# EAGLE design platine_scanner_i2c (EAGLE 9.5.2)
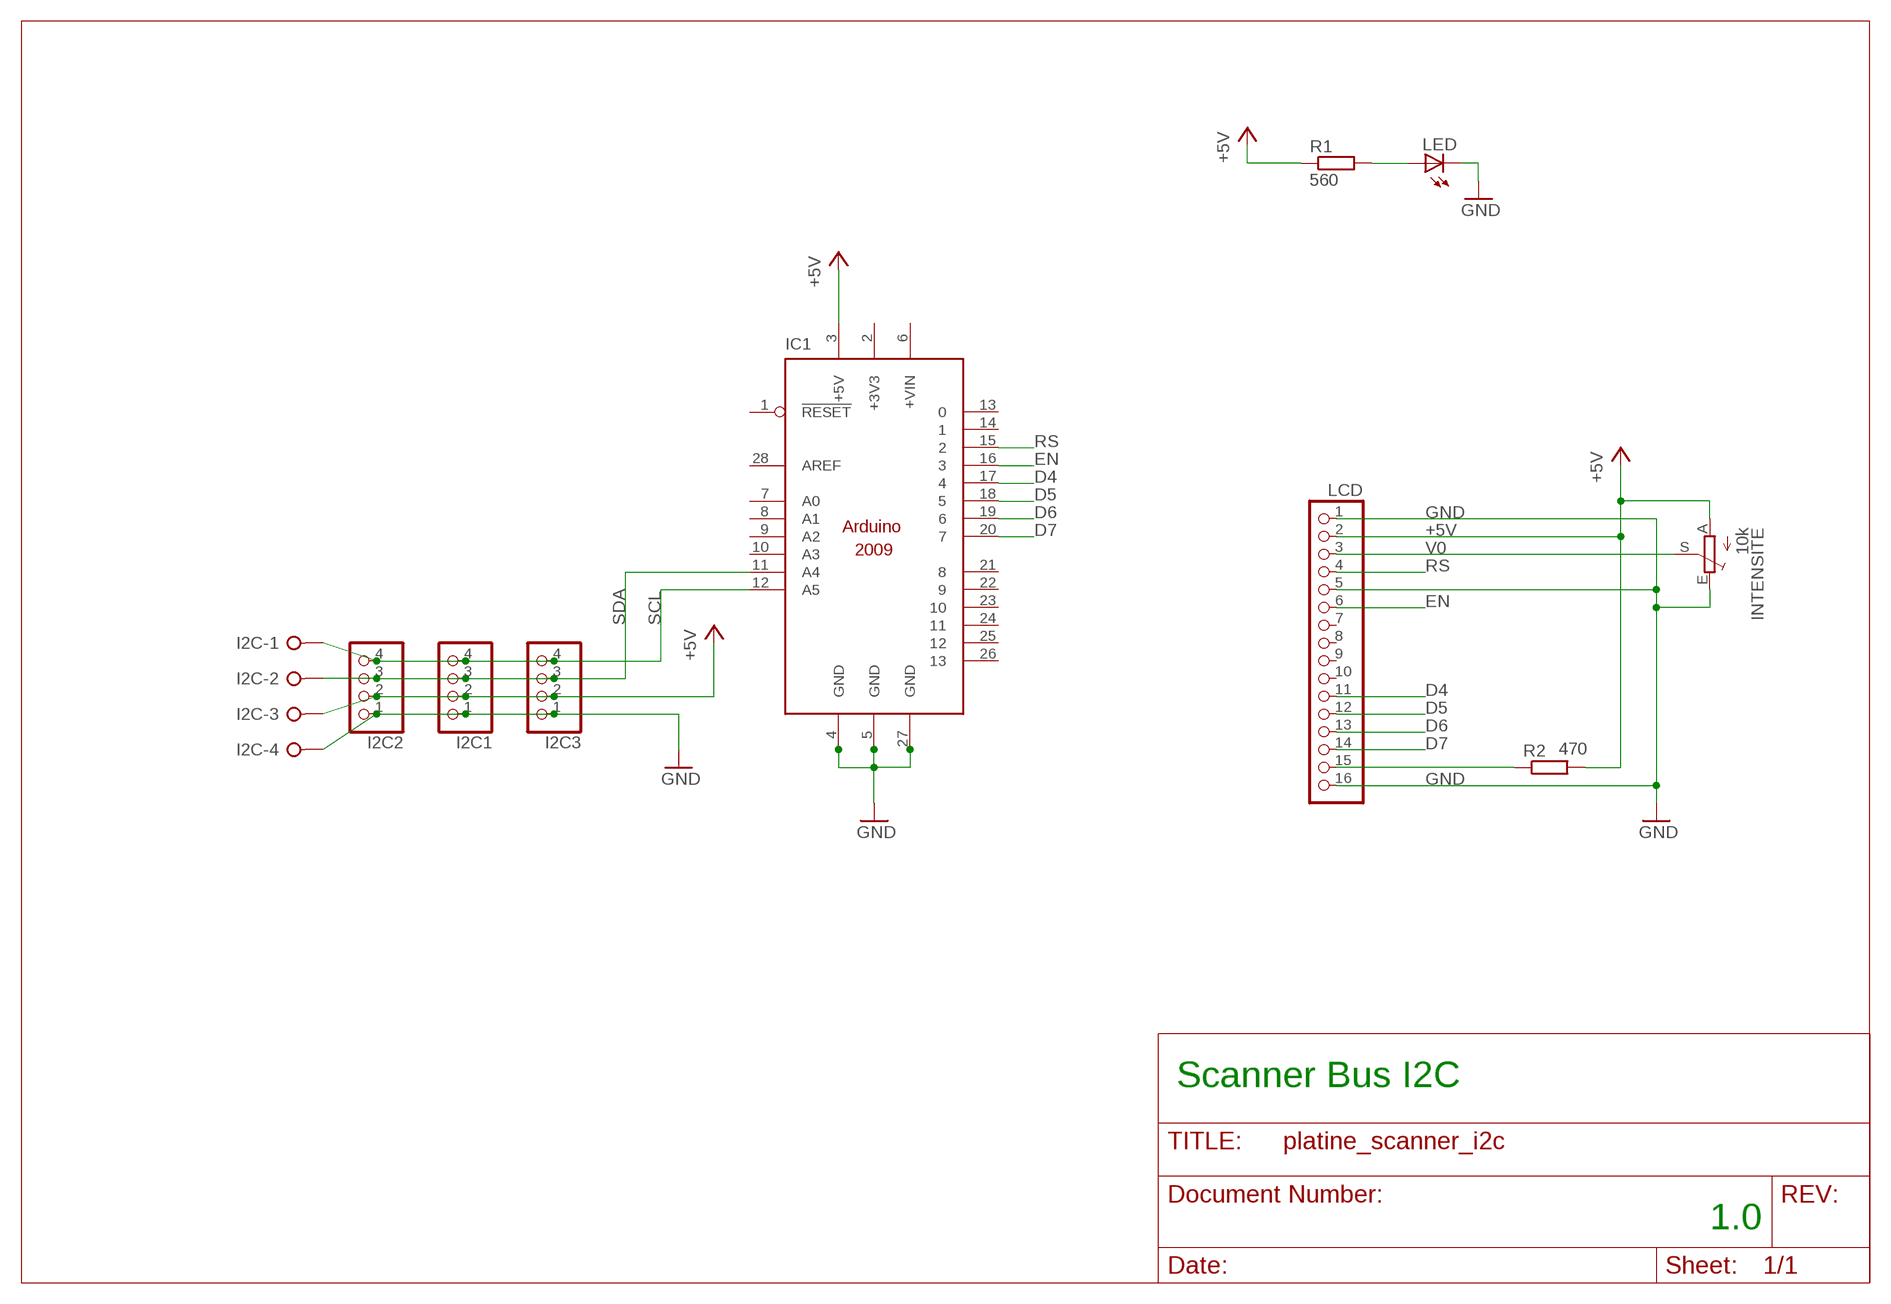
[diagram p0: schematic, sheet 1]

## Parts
I2C  W237-04P  [W237-4P]
I2C1  PINHD-1X4  [1X04]
I2C2  PINHD-1X4  [1X04]
I2C3  PINHD-1X4  [1X04]
IC1  ARDUINO2009_11  [ARDUINO2009_1]
INTENSITE  10k  TRIM_EU-LI10  [LI10]
LCD  PINHD-1X16  [1X16]
LED  LED3MM  [LED3MM]
R1  560  R-EU_0204/7  [0204/7]
R2  470  R-EU_0204/7  [0204/7]

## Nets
+5V: I2C1.2 I2C2.2 I2C3.2 I2C.3 IC1.3(+5V) INTENSITE.A LCD.2 R1.1 R2.2
D4: IC1.17 LCD.11
D5: IC1.18 LCD.12
D6: IC1.19 LCD.13
D7: IC1.20 LCD.14
EN: IC1.16 LCD.6
GND: I2C1.1 I2C2.1 I2C3.1 I2C.4 IC1.4(GND) IC1.5(GND) IC1.27(GND) INTENSITE.E LCD.1 LCD.5 LCD.16 LED.K(C)
N$1: LED.A R1.2
N$15: LCD.15 R2.1
RS: IC1.15 LCD.4
SCL: I2C1.4 I2C2.4 I2C3.4 I2C.1 IC1.12(A5)
SDA: I2C1.3 I2C2.3 I2C3.3 I2C.2 IC1.11(A4)
V0: INTENSITE.S LCD.3
Unconnected: IC1.1(!RESET) IC1.6(+VIN) IC1.7(A0) IC1.8(A1) IC1.9(A2) IC1.10(A3) IC1.13 IC1.14 IC1.21 IC1.22 IC1.23 IC1.24 IC1.25 IC1.26 IC1.28(AREF) LCD.7 LCD.8 LCD.9 LCD.10

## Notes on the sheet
- Scanner Bus I2C
- 1.0

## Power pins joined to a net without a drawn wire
+3V3: IC1.2(+3V3)

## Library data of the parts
I2C = con-wago-508:W237-04P: WAGO SREW CLAMP; OC_FARNELL: unknown; OC_NEWARK: unknown
I2C1-I2C3 = pinhead:PINHD-1X4: PIN HEADER
IC1 = arduino_uno:ARDUINO2009_1: The Arduino Duemilanove ("2009") is a microcontroller board based on the ATmega168 or ATmega328. - 14 digital input/output pins (of which 6 can be used as PWM outputs) - 6 analog inputs, a 16 MHz crystal oscillator - USB connection - power jack - ISP header - reset button It contains everything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
INTENSITE = pot:TRIM_EU-: POTENTIOMETER
LCD = pinhead:PINHD-1X16: PIN HEADER
LED = led:LED: LED
R1 R2 = rcl:R-EU_: RESISTOR, European symbol

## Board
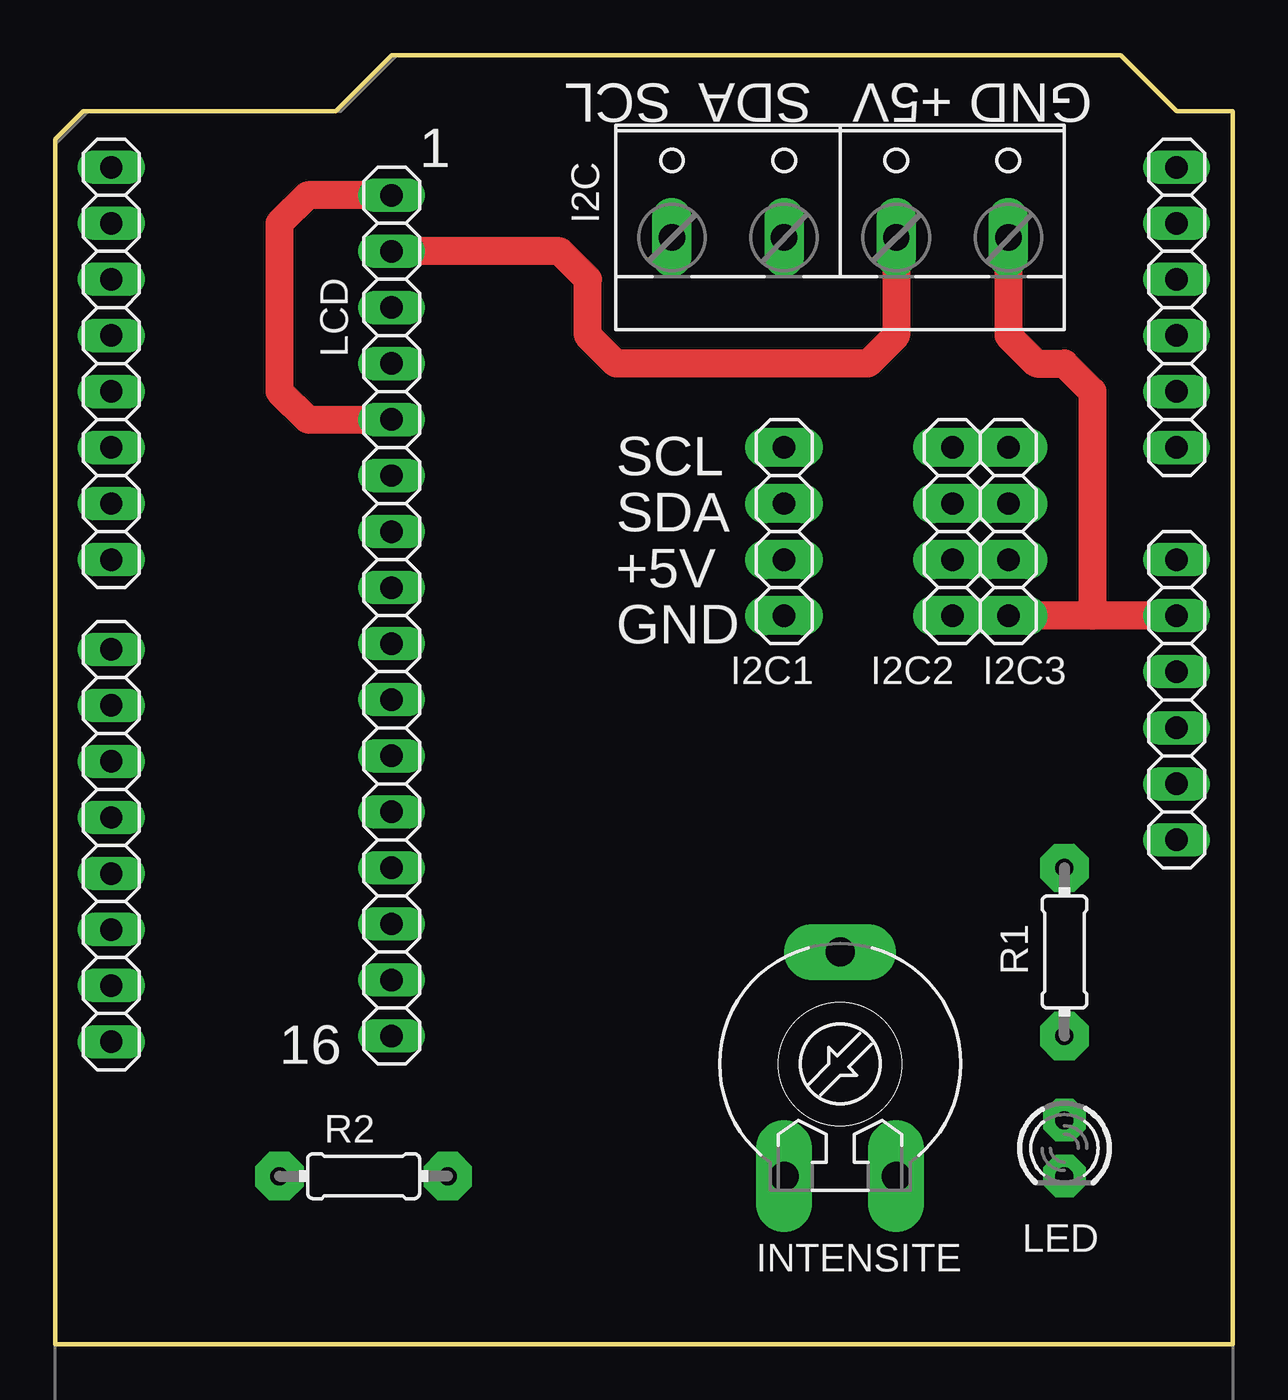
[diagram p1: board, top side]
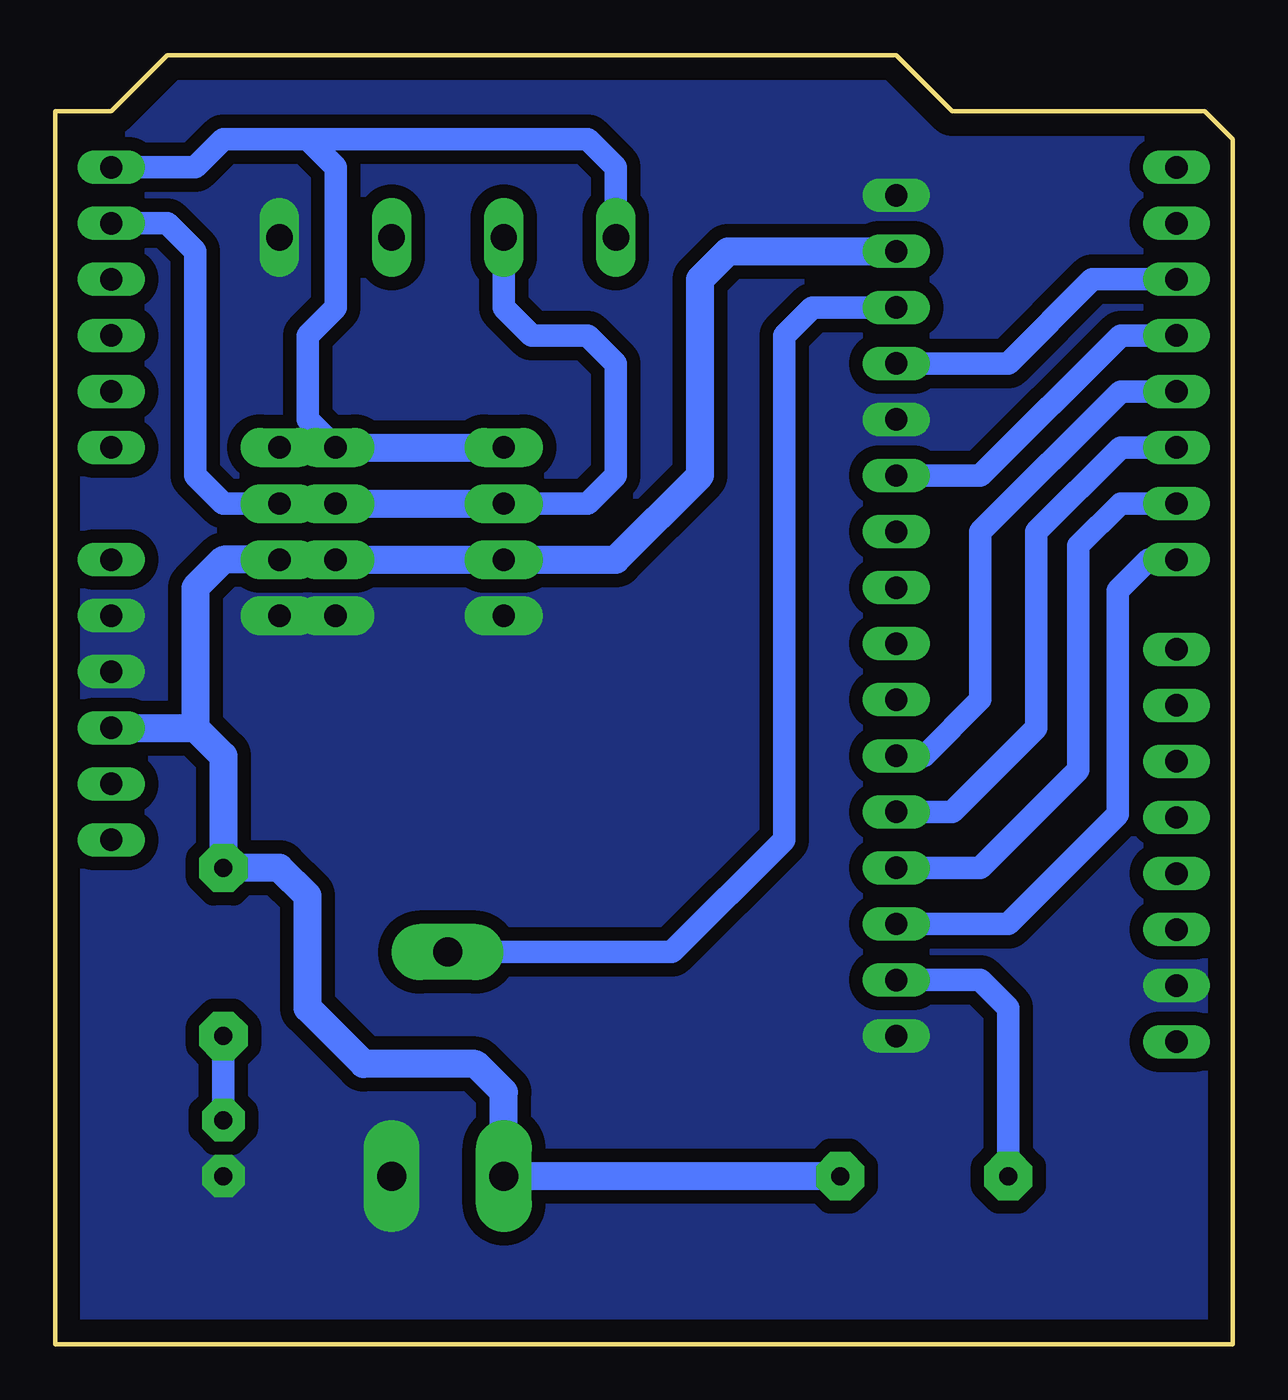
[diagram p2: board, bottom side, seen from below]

Size 53.34 x 58.42 mm. Coordinates in mm from the lower left corner, seen from the top.
Outline: 0,0 0,54.61 1.27,55.88 12.7,55.88 15.24,58.42 48.26,58.42 50.8,55.88 53.34,55.88 53.34,0 0,0
Copper layers (1*16): Top 0.035mm / dielectric 1.5mm / Bottom 0.035mm
Design rules "default": minimum track width 6mil, minimum drill 0.35mm, track to track 6mil, track to pad 6mil, pad to pad 6mil, via to via 6mil, smd to smd 6mil, copper to edge 40mil, drill to drill 6mil, minimum pad ring 10mil, minimum via ring 8mil, stop-mask expansion 4mil, vias tented up to drill 0mil, thermal gap 10mil

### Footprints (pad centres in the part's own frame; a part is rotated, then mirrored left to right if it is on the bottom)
W237-4P = drill 1.194 long: 1 -7.62,-0.635; 2 -2.54,-0.635; 3 2.54,-0.635; 4 7.62,-0.635
1X04 = drill 1.016 pad 1.778 long: 1 -3.81,0; 2 -1.27,0; 3 1.27,0; 4 3.81,0
ARDUINO2009_1 = drill 1.016 long: 1 33.02,2.54; 2 35.56,2.54; 3 38.1,2.54; 4 40.64,2.54; 5 43.18,2.54; 6 45.72,2.54; 7 50.8,2.54; 8 53.34,2.54; 9 55.88,2.54; 10 58.42,2.54; 11 60.96,2.54; 12 63.5,2.54; 13 63.5,50.8; 14 60.96,50.8; 15 58.42,50.8; 16 55.88,50.8; 17 53.34,50.8; 18 50.8,50.8; 19 48.26,50.8; 20 45.72,50.8; 21 41.656,50.8; 22 39.116,50.8; 23 36.576,50.8; 24 34.036,50.8; 25 31.496,50.8; 26 28.956,50.8; 27 26.416,50.8; 28 23.876,50.8
LI10 = drill 1.321 pad 2.54 long: A -2.54,-5.08; E 2.54,-5.08; S 0,5.08
1X16 = drill 1.016 long: 1 -19.05,0; 2 -16.51,0; 3 -13.97,0; 4 -11.43,0; 5 -8.89,0; 6 -6.35,0; 7 -3.81,0; 8 -1.27,0; 9 1.27,0; 10 3.81,0; 11 6.35,0; 12 8.89,0; 13 11.43,0; 14 13.97,0; 15 16.51,0; 16 19.05,0
LED3MM = drill 0.813 pad 1.93 octagon: A -1.27,0; K 1.27,0
0204/7 = drill 0.813 pad 2.184 octagon: 1 -3.81,0; 2 3.81,0

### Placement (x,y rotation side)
I2C  35.56,50.8 0 top
I2C1  33.02,36.83 90 top
I2C2  43.18,36.83 90 top
I2C3  40.64,36.83 90 top
IC1  53.34,-10.16 90 top
INTENSITE  35.56,12.7 0 top
LCD  15.24,33.02 270 top
LED  45.72,8.89 270 top
R1  45.72,17.78 270 top
R2  13.97,7.62 0 top

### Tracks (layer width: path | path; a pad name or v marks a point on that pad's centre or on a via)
+5V
  Top 1.27: I2C.3 38.1,45.72 36.83,44.45 25.4,44.45 24.13,45.72 24.13,48.26 22.86,49.53 LCD.2
  Bottom 1.27: 46.99,27.94 45.72,26.67 R1.1 43.18,21.59 41.91,20.32 41.91,15.24 39.37,12.7 34.29,12.7 33.02,11.43 INTENSITE.A R2.2 | LCD.2 22.86,49.53 24.13,48.26 24.13,39.37 27.94,35.56 I2C1.2 I2C3.2 I2C2.2 45.72,35.56 46.99,34.29 46.99,27.94 | IC1.3 46.99,27.94
D4
  Bottom 1.016: LCD.11 13.97,26.67 11.43,29.21 11.43,36.83 5.08,43.18 IC1.17
D5
  Bottom 1.016: LCD.12 12.7,24.13 8.89,27.94 8.89,36.83 5.08,40.64 IC1.18
D6
  Bottom 1.016: IC1.19 5.08,38.1 6.98,36.2 6.98,26.04 11.43,21.59 LCD.13
D7
  Bottom 1.016: LCD.14 10.16,19.05 5.21,24 5.21,34.16 3.81,35.56 IC1.20
EN
  Bottom 1.016: IC1.16 5.08,45.72 11.43,39.37 LCD.6
GND
  Top 1.27: I2C.4 43.18,45.72 44.45,44.45 45.72,44.45 46.99,43.18 46.99,33.02 I2C2.1 IC1.5 | LCD.5 11.43,41.91 10.16,43.18 10.16,50.8 11.43,52.07 LCD.1
  pour Bottom (isolate 0.61, no thermals): -1.27,58.42 -1.27,-1.27 54.61,-1.27 54.61,58.42
N$1
  Bottom 1.016: R1.2 LED.A
N$15
  Bottom 1.016: LCD.15 11.43,16.51 10.16,15.24 R2.1
RS
  Bottom 1.016: IC1.15 6.35,48.26 10.16,44.45 LCD.4
SCL
  Bottom 1.016: I2C3.4 41.91,41.91 41.91,45.72 40.64,46.99 40.64,53.34 41.91,54.61 | IC1.12 46.99,53.34 45.72,54.61 41.91,54.61 | I2C.1 27.94,53.34 29.21,54.61 41.91,54.61
  Bottom 1.27: I2C1.4 I2C3.4 I2C2.4
SDA
  Bottom 1.016: IC1.11 48.26,50.8 46.99,49.53 46.99,39.37 45.72,38.1 I2C2.3 | I2C.2 33.02,46.99 31.75,45.72 29.21,45.72 27.94,44.45 27.94,39.37 29.21,38.1 I2C1.3
  Bottom 1.27: I2C2.3 I2C3.3 I2C1.3
V0
  Bottom 1.016: INTENSITE.S 25.4,17.78 20.32,22.86 20.32,45.72 19.05,46.99 LCD.3

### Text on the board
tNames: SCL | SDA | +5V | GND | 1 | SCL | SDA | +5V | GND | 16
